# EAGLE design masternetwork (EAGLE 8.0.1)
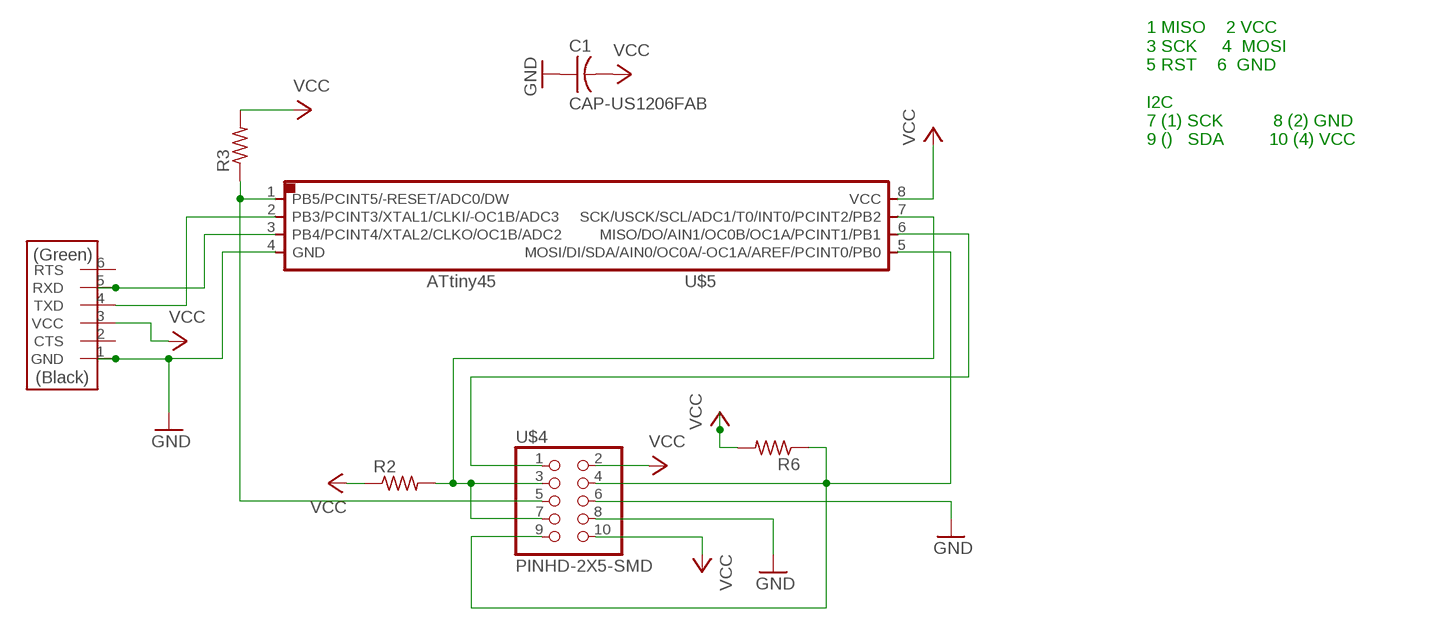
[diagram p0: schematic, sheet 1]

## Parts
C1  CAP-US1206FAB  [C1206FAB]
R2  RES-US1206FAB  [R1206FAB]
R3  RES-US1206FAB  [R1206FAB]
R6  RES-US1206FAB  [R1206FAB]
U$4  PINHD-2X5-SMD  [2X05SMD]
U$5  ATTINY45SI  [SOIC8]
U$6  FTDI-SMD-HEADER  [1X06SMD]

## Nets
GND: C1.1 U$4.6 U$4.8 U$5.4(GND) U$6.1(GND)
N$7: U$4.1 U$5.6(MISO/DO/AIN1/OC0B/OC1A/PCINT1/PB1)
N$8: R6.1 U$4.4 U$4.9 U$5.5(MOSI/DI/SDA/AIN0/OC0A/-OC1A/AREF/PCINT0/PB0)
N$9: R3.1 U$4.5 U$5.1(PB5/PCINT5/-RESET/ADC0/DW)
N$10: R2.2 U$4.3 U$4.7 U$5.7(SCK/USCK/SCL/ADC1/T0/INT0/PCINT2/PB2)
N$11: U$5.3(PB4/PCINT4/XTAL2/CLKO/OC1B/ADC2) U$6.5(RXD)
N$12: U$5.2(PB3/PCINT3/XTAL1/CLKI/-OC1B/ADC3) U$6.4(TXD)
VCC: C1.2 R2.1 R3.2 R6.2 U$4.2 U$4.10 U$5.8(VCC) U$6.3(VCC)
Unconnected: U$6.2(CTS) U$6.6(RTS)

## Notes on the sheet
- 1 MISO    2 VCC
  3 SCK     4  MOSI
  5 RST    6  GND
  
  I2C
  7 (1) SCK          8 (2) GND
  9 ()   SDA         10 (4) VCC

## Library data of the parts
C1 = fab:CAP-US
R2 R3 R6 = fab:RES-US: Resistor (US Symbol)
U$4 = fab:PINHD-2X5-SMD
U$5 = fab:ATTINY45
U$6 = fab:FTDI-SMD-HEADER

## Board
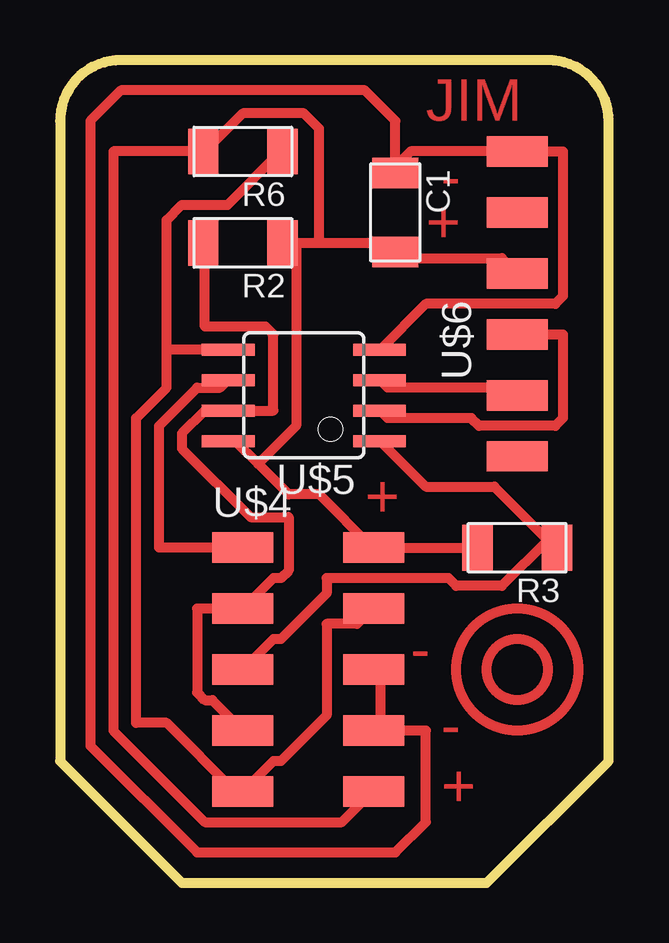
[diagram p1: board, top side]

Size 22.86 x 34.29 mm. Coordinates in mm from the lower left corner, seen from the top.
Outline: 0,31.75 0,5.08 5.08,0 17.78,0 22.86,5.08 22.86,31.75 arc90 20.32,34.29 2.54,34.29 arc90 0,31.75
Copper layers (1*16): Top 0.035mm / dielectric 1.5mm / Bottom 0.035mm
Design rules "default *": minimum track width 16mil, minimum drill 24mil, track to track 16mil, track to pad 16mil, pad to pad 16mil, via to via 16mil, smd to smd 8mil, copper to edge 40mil, drill to drill 8mil, minimum pad ring 10mil, minimum via ring 8mil, stop-mask expansion 4mil, vias tented up to drill 0mil, thermal gap 10mil

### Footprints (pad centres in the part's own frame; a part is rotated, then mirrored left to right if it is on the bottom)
C1206FAB = smd 1.27 x 1.905: 1 -1.651,0; 2 1.651,0
R1206FAB = smd 1.27 x 1.905: 1 -1.651,0; 2 1.651,0
2X05SMD = smd 2.54 x 1.27: 1 -2.54,2.54; 2 2.92,2.54; 3 -2.54,0; 4 2.92,0; 5 -2.54,-2.54; 6 2.92,-2.54; 7 -2.54,-5.08; 8 2.92,-5.08; 9 -2.54,-7.62; 10 2.92,-7.62
SOIC8 = smd 0.5 x 2.2: 1 -1.905,-3.154; 2 -0.645,-3.154; 3 0.625,-3.154; 4 1.895,-3.154; 5 1.905,3.154; 6 0.635,3.154; 7 -0.635,3.154; 8 -1.905,3.154
1X06SMD = smd 2.54 x 1.27: 1 0,6.35; 2 0,3.81; 3 0,1.27; 4 0,-1.27; 5 0,-3.81; 6 0,-6.35

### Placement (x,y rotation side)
C1  13.97,27.94 270 top
R2  7.62,26.67 180 top
R3  19.05,13.97 180 top
R6  7.62,30.48 180 top
U$4  10.16,11.43 0 top
U$5  10.16,20.32 90 top
U$6  19.05,24.13 0 top

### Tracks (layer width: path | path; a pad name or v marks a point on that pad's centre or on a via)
GND
  Top 0.406: U$5.4 13.34,22.23 15.24,24.13 20.64,24.13 20.95,24.45 20.95,30.48 U$6.1 14.61,30.48 13.97,29.84 C1.1 13.97,31.75 12.7,33.02 2.54,33.02 1.27,31.75 1.27,5.71 5.71,1.27 13.97,1.27 15.24,2.54 15.24,6.35 U$4.8 13.34,6.35 13.34,8.89 U$4.6
N$7
  Top 0.406: U$4.1 4.13,13.97 4.13,19.05 5.71,20.64 6.67,20.64 6.99,20.96 U$5.6
N$8
  Top 0.406: 4.44,22.23 4.44,27.62 5.08,28.26 6.99,28.26 9.21,30.48 R6.1 | U$5.5 4.44,22.23 | U$4.4 13.02,11.43 12.38,10.79 11.11,10.79 11.11,6.99 9.21,5.08 8.89,5.08 U$4.9 7.3,3.81 4.44,6.67 3.17,6.67 3.17,19.37 4.44,20.64 4.44,22.23
N$9
  Top 0.406: 20.32,14.29 18.1,16.51 15.24,16.51 13.34,18.41 U$5.1 | 20.32,14.29 20.64,13.97 R3.1 20.32,14.29 | U$4.5 8.89,10.16 9.21,10.16 11.11,12.07 11.11,12.7 16.19,12.7 16.51,12.38 18.41,12.38 20.32,14.29
N$10
  Top 0.406: U$4.7 6.35,7.62 6.03,7.62 5.71,7.94 5.71,11.43 U$4.3 8.89,12.7 9.21,12.7 9.53,13.02 9.53,15.24 7.94,15.24 5.08,18.1 5.08,18.73 6.03,19.68 U$5.7 8.89,19.68 8.89,22.86 8.57,23.18 6.03,23.18 6.03,26.67 R2.2
N$11
  Top 0.406: U$6.5 18.73,20.64 13.65,20.64 13.34,20.96 U$5.3
N$12
  Top 0.406: U$6.4 20.95,22.86 20.95,19.37 20.64,19.05 17.46,19.05 17.14,19.37 13.65,19.37 13.34,19.68 U$5.2
VCC
  Top 0.406: R3.2 U$4.2 13.02,13.97 10.79,16.19 9.53,16.19 8.26,17.46 | 8.26,17.46 7.3,18.41 U$5.8 | 9.84,26.67 R2.1 9.53,26.67 | 9.84,26.67 10.79,26.67 | 10.79,26.67 13.65,26.67 13.97,26.35 C1.2 13.97,26.04 18.41,26.04 U$6.3 | 10.79,26.67 10.79,31.43 10.16,32.07 7.62,32.07 6.03,30.48 R6.2 2.22,30.48 2.22,6.35 6.03,2.54 11.75,2.54 13.02,3.81 U$4.10 | 8.26,17.46 9.84,19.05 9.84,26.67
(copper drawn outside any net)
  shapes: Top circle x2

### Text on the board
Top: JIM | - | + | + | - | - | +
